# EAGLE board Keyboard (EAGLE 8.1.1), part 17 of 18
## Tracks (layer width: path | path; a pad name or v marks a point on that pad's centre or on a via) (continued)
S$17665
  Bottom 0: 136.24,76.22 136.19,76.17
S$17666
  Bottom 0: 136.19,76.17 136.01,75.89
S$17667
  Bottom 0: 136.01,75.89 135.93,75.58
S$17668
  Bottom 0: 135.93,75.58 135.93,75.25
S$17669
  Bottom 0: 135.93,75.25 136.01,74.94
S$17670
  Bottom 0: 136.01,74.94 136.11,74.79
S$17671
  Bottom 0: 136.11,74.79 133.86,77.04
S$17672
  Bottom 0: 133.86,77.04 133.81,77.09
S$17673
  Bottom 0: 133.81,77.09 133.75,77.12
S$17674
  Bottom 0: 133.75,77.12 133.68,77.15
S$17675
  Bottom 0: 133.68,77.15 133.61,77.17
S$17676
  Bottom 0: 133.61,77.17 133.55,77.17
S$17677
  Bottom 0: 133.55,77.17 123.08,77.17
S$17678
  Bottom 0: 123.08,77.17 123.01,77.17
S$17679
  Bottom 0: 123.01,77.17 122.94,77.15
S$17680
  Bottom 0: 122.94,77.15 122.88,77.13
S$17681
  Bottom 0: 122.88,77.13 122.82,77.09
S$17682
  Bottom 0: 122.82,77.09 122.77,77.05
S$17683
  Bottom 0: 122.77,77.05 120.27,74.55
S$17684
  Bottom 0: 120.27,74.55 118.87,74.55
S$17685
  Bottom 0: 131.47,79.17 131.77,79.23
S$17686
  Bottom 0: 131.77,79.23 132.03,79.39
S$17687
  Bottom 0: 132.03,79.39 132.24,79.61
S$17688
  Bottom 0: 132.24,79.61 132.37,79.88
S$17689
  Bottom 0: 132.37,79.88 132.41,80.18
S$17690
  Bottom 0: 132.41,80.18 132.37,80.48
S$17691
  Bottom 0: 132.37,80.48 132.24,80.75
S$17692
  Bottom 0: 132.24,80.75 132.03,80.97
S$17693
  Bottom 0: 132.03,80.97 131.77,81.12
S$17694
  Bottom 0: 131.77,81.12 131.47,81.19
S$17695
  Bottom 0: 131.47,81.19 131.17,81.17
S$17696
  Bottom 0: 131.17,81.17 130.89,81.06
S$17697
  Bottom 0: 130.89,81.06 130.65,80.87
S$17698
  Bottom 0: 130.65,80.87 130.48,80.62
S$17699
  Bottom 0: 130.48,80.62 130.39,80.33
S$17700
  Bottom 0: 130.39,80.33 130.39,80.03
S$17701
  Bottom 0: 130.39,80.03 130.48,79.74
S$17702
  Bottom 0: 130.48,79.74 130.65,79.49
S$17703
  Bottom 0: 130.65,79.49 130.89,79.3
S$17704
  Bottom 0: 130.89,79.3 131.17,79.19
S$17705
  Bottom 0: 131.17,79.19 131.47,79.17
S$17706
  Bottom 0: 125.75,79.83 126.1,79.89
S$17707
  Bottom 0: 126.1,79.89 126.41,80.04
S$17708
  Bottom 0: 126.41,80.04 126.68,80.26
S$17709
  Bottom 0: 126.68,80.26 126.89,80.55
S$17710
  Bottom 0: 126.89,80.55 127.02,80.87
S$17711
  Bottom 0: 127.02,80.87 127.06,81.22
S$17712
  Bottom 0: 127.06,81.22 127.02,81.56
S$17713
  Bottom 0: 127.02,81.56 126.89,81.89
S$17714
  Bottom 0: 126.89,81.89 126.68,82.17
S$17715
  Bottom 0: 126.68,82.17 126.41,82.39
S$17716
  Bottom 0: 126.41,82.39 126.1,82.55
S$17717
  Bottom 0: 126.1,82.55 125.75,82.61
S$17718
  Bottom 0: 125.75,82.61 125.4,82.59
S$17719
  Bottom 0: 125.4,82.59 125.07,82.48
S$17720
  Bottom 0: 125.07,82.48 124.78,82.29
S$17721
  Bottom 0: 124.78,82.29 124.54,82.04
S$17722
  Bottom 0: 124.54,82.04 124.37,81.73
S$17723
  Bottom 0: 124.37,81.73 124.28,81.39
S$17724
  Bottom 0: 124.28,81.39 124.28,81.04
S$17725
  Bottom 0: 124.28,81.04 124.37,80.7
S$17726
  Bottom 0: 124.37,80.7 124.54,80.39
S$17727
  Bottom 0: 124.54,80.39 124.78,80.14
S$17728
  Bottom 0: 124.78,80.14 125.07,79.95
S$17729
  Bottom 0: 125.07,79.95 125.4,79.84
S$17730
  Bottom 0: 125.4,79.84 125.75,79.83
S$17731
  Bottom 0: 121.86,81.47 122.3,81.52
S$17732
  Bottom 0: 122.3,81.52 122.73,81.64
S$17733
  Bottom 0: 122.73,81.64 123.13,81.86
S$17734
  Bottom 0: 123.13,81.86 123.47,82.14
S$17735
  Bottom 0: 123.47,82.14 123.76,82.49
S$17736
  Bottom 0: 123.76,82.49 123.97,82.88
S$17737
  Bottom 0: 123.97,82.88 124.1,83.31
S$17738
  Bottom 0: 124.1,83.31 124.14,83.76
S$17739
  Bottom 0: 124.14,83.76 124.1,84.2
S$17740
  Bottom 0: 124.1,84.2 123.97,84.63
S$17741
  Bottom 0: 123.97,84.63 123.76,85.03
S$17742
  Bottom 0: 123.76,85.03 123.47,85.37
S$17743
  Bottom 0: 123.47,85.37 123.13,85.66
S$17744
  Bottom 0: 123.13,85.66 122.73,85.87
S$17745
  Bottom 0: 122.73,85.87 122.3,86
S$17746
  Bottom 0: 122.3,86 121.86,86.04
S$17747
  Bottom 0: 121.86,86.04 121.41,86
S$17748
  Bottom 0: 121.41,86 120.98,85.87
S$17749
  Bottom 0: 120.98,85.87 120.59,85.66
S$17750
  Bottom 0: 120.59,85.66 120.24,85.37
S$17751
  Bottom 0: 120.24,85.37 119.96,85.03
S$17752
  Bottom 0: 119.96,85.03 119.74,84.63
S$17753
  Bottom 0: 119.74,84.63 119.61,84.2
S$17754
  Bottom 0: 119.61,84.2 119.57,83.76
S$17755
  Bottom 0: 119.57,83.76 119.61,83.31
S$17756
  Bottom 0: 119.61,83.31 119.74,82.88
S$17757
  Bottom 0: 119.74,82.88 119.96,82.49
S$17758
  Bottom 0: 119.96,82.49 120.24,82.14
S$17759
  Bottom 0: 120.24,82.14 120.59,81.86
S$17760
  Bottom 0: 120.59,81.86 120.98,81.64
S$17761
  Bottom 0: 120.98,81.64 121.41,81.52
S$17762
  Bottom 0: 121.41,81.52 121.86,81.47
S$17763
  Bottom 0: 131.47,86.79 131.77,86.86
S$17764
  Bottom 0: 131.77,86.86 132.03,87.01
S$17765
  Bottom 0: 132.03,87.01 132.24,87.23
S$17766
  Bottom 0: 132.24,87.23 132.37,87.5
S$17767
  Bottom 0: 132.37,87.5 132.41,87.8
S$17768
  Bottom 0: 132.41,87.8 132.37,88.1
S$17769
  Bottom 0: 132.37,88.1 132.24,88.37
S$17770
  Bottom 0: 132.24,88.37 132.03,88.59
S$17771
  Bottom 0: 132.03,88.59 131.77,88.75
S$17772
  Bottom 0: 131.77,88.75 131.47,88.81
S$17773
  Bottom 0: 131.47,88.81 131.17,88.79
S$17774
  Bottom 0: 131.17,88.79 130.89,88.68
S$17775
  Bottom 0: 130.89,88.68 130.65,88.49
S$17776
  Bottom 0: 130.65,88.49 130.48,88.24
S$17777
  Bottom 0: 130.48,88.24 130.39,87.95
S$17778
  Bottom 0: 130.39,87.95 130.39,87.65
S$17779
  Bottom 0: 130.39,87.65 130.48,87.36
S$17780
  Bottom 0: 130.48,87.36 130.65,87.11
S$17781
  Bottom 0: 130.65,87.11 130.89,86.92
S$17782
  Bottom 0: 130.89,86.92 131.17,86.81
S$17783
  Bottom 0: 131.17,86.81 131.47,86.79
S$17784
  Bottom 0: 174.03,75.35 172.15,77.23
S$17785
  Bottom 0: 172.15,77.23 172.09,77.27
S$17786
  Bottom 0: 172.09,77.27 172.03,77.31
S$17787
  Bottom 0: 172.03,77.31 171.97,77.34
S$17788
  Bottom 0: 171.97,77.34 171.91,77.36
S$17789
  Bottom 0: 171.91,77.36 171.83,77.36
S$17790
  Bottom 0: 171.83,77.36 168.25,77.36
S$17791
  Bottom 0: 168.25,77.36 165.01,80.6
S$17792
  Bottom 0: 165.01,80.6 165.12,80.87
S$17793
  Bottom 0: 165.12,80.87 165.16,81.22
S$17794
  Bottom 0: 165.16,81.22 165.12,81.56
S$17795
  Bottom 0: 165.12,81.56 164.99,81.89
S$17796
  Bottom 0: 164.99,81.89 164.78,82.17
S$17797
  Bottom 0: 164.78,82.17 164.51,82.39
S$17798
  Bottom 0: 164.51,82.39 164.2,82.55
S$17799
  Bottom 0: 164.2,82.55 163.85,82.61
S$17800
  Bottom 0: 163.85,82.61 163.5,82.59
S$17801
  Bottom 0: 163.5,82.59 163.17,82.48
S$17802
  Bottom 0: 163.17,82.48 162.88,82.29
S$17803
  Bottom 0: 162.88,82.29 162.64,82.04
S$17804
  Bottom 0: 162.64,82.04 162.56,81.9
S$17805
  Bottom 0: 162.56,81.9 162.56,81.99
S$17806
  Bottom 0: 162.56,81.99 162.88,82.31
S$17807
  Bottom 0: 162.88,82.31 162.94,82.38
S$17808
  Bottom 0: 162.94,82.38 162.99,82.45
S$17809
  Bottom 0: 162.99,82.45 163.03,82.53
S$17810
  Bottom 0: 163.03,82.53 163.04,82.62
S$17811
  Bottom 0: 163.04,82.62 163.05,82.71
S$17812
  Bottom 0: 163.05,82.71 163.05,87.58
S$17813
  Bottom 0: 163.05,87.58 163.04,87.67
S$17814
  Bottom 0: 163.04,87.67 163.03,87.76
S$17815
  Bottom 0: 163.03,87.76 162.99,87.84
S$17816
  Bottom 0: 162.99,87.84 162.94,87.92
S$17817
  Bottom 0: 162.94,87.92 162.88,87.98
S$17818
  Bottom 0: 162.88,87.98 162.33,88.54
S$17819
  Bottom 0: 162.33,88.54 162.37,88.84
S$17820
  Bottom 0: 162.37,88.84 162.32,89.16
S$17821
  Bottom 0: 162.32,89.16 162.19,89.46
S$17822
  Bottom 0: 162.19,89.46 162.01,89.65
S$17823
  Bottom 0: 162.01,89.65 176.59,89.65
S$17824
  Bottom 0: 176.59,89.65 176.59,87.95
S$17825
  Bottom 0: 176.59,87.95 176.6,87.87
S$17826
  Bottom 0: 176.6,87.87 176.64,87.8
S$17827
  Bottom 0: 176.64,87.8 176.7,87.74
S$17828
  Bottom 0: 176.7,87.74 176.77,87.7
S$17829
  Bottom 0: 176.77,87.7 176.85,87.69
S$17830
  Bottom 0: 176.85,87.69 177.24,87.69
S$17831
  Bottom 0: 177.24,87.69 174.62,85.08
S$17832
  Bottom 0: 174.62,85.08 174.58,85.03
S$17833
  Bottom 0: 174.58,85.03 174.54,84.97
S$17834
  Bottom 0: 174.54,84.97 174.51,84.91
S$17835
  Bottom 0: 174.51,84.91 174.5,84.84
S$17836
  Bottom 0: 174.5,84.84 174.49,84.77
S$17837
  Bottom 0: 174.49,84.77 174.49,76.36
S$17838
  Bottom 0: 174.49,76.36 174.29,76.17
S$17839
  Bottom 0: 174.29,76.17 174.12,75.89
S$17840
  Bottom 0: 174.12,75.89 174.03,75.58
S$17841
  Bottom 0: 174.03,75.58 174.03,75.35
S$17842
  Bottom 0: 169.24,78.25 169.76,78.25
S$17843
  Bottom 0: 169.76,78.25 170.27,78.34
S$17844
  Bottom 0: 170.27,78.34 170.76,78.5
S$17845
  Bottom 0: 170.76,78.5 171.21,78.75
S$17846
  Bottom 0: 171.21,78.75 171.62,79.07
S$17847
  Bottom 0: 171.62,79.07 171.98,79.45
S$17848
  Bottom 0: 171.98,79.45 172.26,79.88
S$17849
  Bottom 0: 172.26,79.88 172.47,80.36
S$17850
  Bottom 0: 172.47,80.36 172.6,80.86
S$17851
  Bottom 0: 172.6,80.86 172.64,81.37
S$17852
  Bottom 0: 172.64,81.37 172.6,81.89
S$17853
  Bottom 0: 172.6,81.89 172.47,82.39
S$17854
  Bottom 0: 172.47,82.39 172.26,82.87
S$17855
  Bottom 0: 172.26,82.87 171.98,83.3
S$17856
  Bottom 0: 171.98,83.3 171.62,83.68
S$17857
  Bottom 0: 171.62,83.68 171.21,84
S$17858
  Bottom 0: 171.21,84 170.76,84.24
S$17859
  Bottom 0: 170.76,84.24 170.27,84.41
S$17860
  Bottom 0: 170.27,84.41 169.76,84.5
S$17861
  Bottom 0: 169.76,84.5 169.24,84.5
S$17862
  Bottom 0: 169.24,84.5 168.74,84.41
S$17863
  Bottom 0: 168.74,84.41 168.24,84.24
S$17864
  Bottom 0: 168.24,84.24 167.79,84
S$17865
  Bottom 0: 167.79,84 167.38,83.68
S$17866
  Bottom 0: 167.38,83.68 167.03,83.3
S$17867
  Bottom 0: 167.03,83.3 166.74,82.87
S$17868
  Bottom 0: 166.74,82.87 166.53,82.39
S$17869
  Bottom 0: 166.53,82.39 166.41,81.89
S$17870
  Bottom 0: 166.41,81.89 166.37,81.37
S$17871
  Bottom 0: 166.37,81.37 166.41,80.86
S$17872
  Bottom 0: 166.41,80.86 166.53,80.36
S$17873
  Bottom 0: 166.53,80.36 166.74,79.88
S$17874
  Bottom 0: 166.74,79.88 167.03,79.45
S$17875
  Bottom 0: 167.03,79.45 167.38,79.07
S$17876
  Bottom 0: 167.38,79.07 167.79,78.75
S$17877
  Bottom 0: 167.79,78.75 168.24,78.5
S$17878
  Bottom 0: 168.24,78.5 168.74,78.34
S$17879
  Bottom 0: 168.74,78.34 169.24,78.25
S$17880
  Bottom 0: 322.05,75.88 321.98,76.03
S$17881
  Bottom 0: 321.98,76.03 321.77,76.29
S$17882
  Bottom 0: 321.77,76.29 321.51,76.48
S$17883
  Bottom 0: 321.51,76.48 321.2,76.58
S$17884
  Bottom 0: 321.2,76.58 320.88,76.6
S$17885
  Bottom 0: 320.88,76.6 320.56,76.54
S$17886
  Bottom 0: 320.56,76.54 320.27,76.39
S$17887
  Bottom 0: 320.27,76.39 320.09,76.22
S$17888
  Bottom 0: 320.09,76.22 320.09,79.82
S$17889
  Bottom 0: 320.09,79.82 320.24,79.81
S$17890
  Bottom 0: 320.24,79.81 320.55,79.86
S$17891
  Bottom 0: 320.55,79.86 320.65,79.83
S$17892
  Bottom 0: 320.65,79.83 321,79.81
S$17893
  Bottom 0: 321,79.81 321.35,79.87
S$17894
  Bottom 0: 321.35,79.87 321.66,80.02
S$17895
  Bottom 0: 321.66,80.02 321.93,80.25
S$17896
  Bottom 0: 321.93,80.25 322.05,80.41
S$17897
  Bottom 0: 322.05,80.41 322.05,75.88
S$17898
  Bottom 0: 223.34,79.41 222.16,80.6
S$17899
  Bottom 0: 222.16,80.6 222.27,80.87
S$17900
  Bottom 0: 222.27,80.87 222.31,81.22
S$17901
  Bottom 0: 222.31,81.22 222.27,81.56
S$17902
  Bottom 0: 222.27,81.56 222.14,81.89
S$17903
  Bottom 0: 222.14,81.89 221.93,82.17
S$17904
  Bottom 0: 221.93,82.17 221.66,82.39
S$17905
  Bottom 0: 221.66,82.39 221.35,82.55
S$17906
  Bottom 0: 221.35,82.55 221,82.61
S$17907
  Bottom 0: 221,82.61 220.65,82.59
S$17908
  Bottom 0: 220.65,82.59 220.32,82.48
S$17909
  Bottom 0: 220.32,82.48 220.03,82.29
S$17910
  Bottom 0: 220.03,82.29 219.79,82.04
S$17911
  Bottom 0: 219.79,82.04 219.79,82.06
S$17912
  Bottom 0: 219.79,82.06 220.03,82.31
S$17913
  Bottom 0: 220.03,82.31 220.09,82.38
S$17914
  Bottom 0: 220.09,82.38 220.14,82.45
S$17915
  Bottom 0: 220.14,82.45 220.18,82.53
S$17916
  Bottom 0: 220.18,82.53 220.19,82.62
S$17917
  Bottom 0: 220.19,82.62 220.2,82.71
S$17918
  Bottom 0: 220.2,82.71 220.2,87.58
S$17919
  Bottom 0: 220.2,87.58 220.19,87.66
S$17920
  Bottom 0: 220.19,87.66 220.18,87.75
S$17921
  Bottom 0: 220.18,87.75 220.14,87.84
S$17922
  Bottom 0: 220.14,87.84 220.09,87.91
S$17923
  Bottom 0: 220.09,87.91 220.03,87.98
S$17924
  Bottom 0: 220.03,87.98 219.48,88.54
S$17925
  Bottom 0: 219.48,88.54 219.52,88.84
S$17926
  Bottom 0: 219.52,88.84 219.49,89.05
S$17927
  Bottom 0: 219.49,89.05 226.21,82.32
S$17928
  Bottom 0: 226.21,82.32 226.21,81.09
S$17929
  Bottom 0: 226.21,81.09 226.14,81.06
S$17930
  Bottom 0: 226.14,81.06 225.91,80.88
S$17931
  Bottom 0: 225.91,80.88 225.74,80.63
S$17932
  Bottom 0: 225.74,80.63 225.64,80.34
S$17933
  Bottom 0: 225.64,80.34 225.64,80.03
S$17934
  Bottom 0: 225.64,80.03 225.74,79.74
S$17935
  Bottom 0: 225.74,79.74 225.91,79.49
S$17936
  Bottom 0: 225.91,79.49 226.01,79.41
S$17937
  Bottom 0: 226.01,79.41 223.34,79.41
S$17938
  Bottom 0.635: 284.09,74.83 284.09,60.85
S$17939
  Bottom 0.635: 284.09,60.85 291.67,53.27
S$17940
  Bottom 0.635: 276.67,22.46 276.67,23.03
S$17941
  Bottom 0.635: 284.99,22.81 284.99,15.92
S$17942
  Bottom 0.635: 284.99,15.92 283.31,14.24
S$17943
  Bottom 0.635: 283.31,14.24 282.44,14.24
S$17944
  Bottom 0.635: 282.44,14.24 276.67,20.02
S$17945
  Bottom 0.635: 276.67,20.02 276.67,22.46
S$17946
  Bottom 0.635: 275.4,22.46 276.67,22.46
S$17947
  Bottom 0.635: 275.4,22.46 275.4,21.32
S$17948
  Bottom 0.635: 275.4,23.03 275.4,22.46
S$17949
  Bottom 0.635: 274.13,23.03 274.13,21.32
S$17950
  Bottom 0.635: 274.13,21.32 275.4,21.32
S$17951
  Bottom 0.635: 289.13,38.03 287.6,39.56
S$17952
  Bottom 0.635: 287.6,39.56 285.93,39.56
S$17953
  Bottom 0.635: 285.93,39.56 285.14,38.78
S$17954
  Bottom 0.635: 285.14,38.78 285.14,35.23
S$17955
  Bottom 0.635: 285.14,35.23 286.46,33.91
S$17956
  Bottom 0.635: 286.46,33.91 286.46,24.28
S$17957
  Bottom 0.635: 286.46,24.28 284.99,22.81
S$17958
  Bottom 0.635: 291.67,53.27 291.81,53.13
S$17959
  Bottom 0.635: 291.81,53.13 291.81,40.71
S$17960
  Bottom 0.635: 291.81,40.71 289.13,38.03
S$17961
  Bottom 0.635: 284.09,74.83 285.37,74.83
S$17962
  Bottom 0.635: 283.78,74.83 284.09,74.83
S$17963
  Bottom 0.635: 289.88,88.52 289.88,85.48
S$17964
  Bottom 0.635: 289.88,85.48 287.82,83.42
S$17965
  Bottom 0.635: 285.37,74.83 285.37,80.97
S$17966
  Bottom 0.635: 285.37,80.97 287.82,83.42
S$17967
  Bottom 0.381: 23.05,62.84 23.05,58
S$17968
  Bottom 0.381: 23.05,58 21.43,56.38
S$17969
  Bottom 0.381: 21.43,56.38 21.43,36.5
S$17970
  Bottom 0.381: 21.43,36.5 19.45,34.52
S$17971
  Bottom 0.381: 19.45,34.52 19.45,31.01
S$17972
  Bottom 0.381: 19.45,31.01 23.27,27.18
S$17973
  Bottom 0.381: 23.27,27.18 23.27,24.07
S$17974
  Bottom 0.381: 11.37,81.21 23.05,69.53
S$17975
  Bottom 0.381: 23.05,69.53 23.05,62.84
S$17976
  Bottom 0.381: 30.31,62.84 23.05,62.84
S$17977
  Bottom 0.381: 230.44,62.16 217.85,62.16
S$17978
  Bottom 0.381: 217.85,62.16 211.53,68.49
S$17979
  Bottom 0.381: 211.53,68.49 205.24,68.49
S$17980
  Bottom 0.381: 205.24,68.49 198.23,75.5
S$17981
  Bottom 0.381: 198.23,75.5 198.23,78.82
S$17982
  Bottom 0.381: 198.23,78.82 195.58,81.46
S$17983
  Bottom 0.381: 195.58,81.46 195.58,84.68
S$17984
  Bottom 0.381: 195.58,84.68 198.04,87.14
S$17985
  Bottom 0.381: 198.04,87.14 198.04,89.98
S$17986
  Bottom 0.381: 198.04,89.98 197.93,90.09
S$17987
  Bottom 0.381: 197.93,90.09 195.67,90.09
S$17988
  Bottom 0.381: 195.67,90.09 186.8,81.22
S$17989
  Bottom 0.381: 186.8,81.22 182.82,81.22
S$17990
  Bottom 0.381: 225.09,10.39 243.96,29.27
S$17991
  Bottom 0.381: 243.96,29.27 243.96,50.19
S$17992
  Bottom 0.381: 243.96,50.19 231.99,62.16
S$17993
  Bottom 0.381: 231.99,62.16 230.44,62.16
S$17994
  Bottom 0.381: 225.09,10.39 224.25,11.23
S$17995
  Bottom 0.381: 224.25,11.23 219.46,11.23
S$17996
  Bottom 0.381: 219.46,11.23 206.63,24.07
S$17997
  Bottom 0.381: 228.06,5.01 228.06,7.42
S$17998
  Bottom 0.381: 228.06,7.42 225.09,10.39
S$17999
  Bottom 0.381: 101.85,43.11 101.85,49.98
S$18000
  Bottom 0.381: 101.85,49.98 94.96,56.87
S$18001
  Bottom 0.381: 94.96,56.87 90.32,56.87
S$18002
  Bottom 0.381: 90.32,56.87 87.39,59.8
S$18003
  Bottom 0.381: 206.63,24.07 208.01,25.45
S$18004
  Bottom 0.381: 208.01,25.45 208.01,41.25
S$18005
  Bottom 0.381: 208.01,41.25 201.14,48.12
S$18006
  Bottom 0.381: 30.42,81.21 24.39,81.21
S$18007
  Bottom 0.381: 24.39,81.21 22.5,79.33
S$18008
  Bottom 0.381: 22.5,79.33 22.5,77.87
S$18009
  Bottom 0.381: 22.5,77.87 25.14,75.23
S$18010
  Bottom 0.381: 25.14,75.23 25.14,68.47
S$18011
  Bottom 0.381: 25.14,68.47 29.97,63.64
S$18012
  Bottom 0.381: 29.97,63.64 29.98,63.65
S$18013
  Bottom 0.381: 29.98,63.65 30.64,63.65
S$18014
  Bottom 0.381: 30.64,63.65 31.11,63.18
S$18015
  Bottom 0.381: 31.11,63.18 31.11,62.51
S$18016
  Bottom 0.381: 31.11,62.51 31.1,62.51
S$18017
  Bottom 0.381: 31.1,62.51 31.3,62.3
S$18018
  Bottom 0.381: 31.3,62.3 33.06,62.3
S$18019
  Bottom 0.381: 33.06,62.3 41.18,54.18
S$18020
  Bottom 0.381: 41.18,54.18 40.9,53.9
S$18021
  Bottom 0.381: 40.9,53.9 40.9,49.1
S$18022
  Bottom 0.381: 40.9,49.1 36.84,45.04
S$18023
  Bottom 0.381: 36.84,45.04 36.84,39.84
S$18024
  Bottom 0.381: 36.84,39.84 46.75,29.93
S$18025
  Bottom 0.381: 46.75,29.93 50.49,29.93
S$18026
  Bottom 0.381: 50.49,29.93 54.23,26.2
S$18027
  Bottom 0.381: 54.23,26.2 54.23,24.07
S$18028
  Bottom 0.381: 41.18,54.18 43.28,56.28
S$18029
  Bottom 0.381: 43.28,56.28 72.4,56.28
S$18030
  Bottom 0.381: 72.4,56.28 74.52,58.39
S$18031
  Bottom 0.381: 248.65,36.62 248.65,19.02
S$18032
  Bottom 0.381: 248.65,19.02 245.54,15.91
S$18033
  Bottom 0.381: 245.54,15.91 245.54,11.47
S$18034
  Bottom 0.381: 245.54,11.47 246.21,10.8
S$18035
  Bottom 0.381: 246.21,10.8 248.34,10.8
S$18036
  Bottom 0.381: 248.34,10.8 251.88,7.26
S$18037
  Bottom 0.381: 251.88,7.26 251.88,5.01
S$18038
  Bottom 0.381: 258.57,55.84 248.65,45.92
S$18039
  Bottom 0.381: 248.65,45.92 248.65,36.62
S$18040
  Bottom 0.381: 258.57,55.84 261.87,52.54
S$18041
  Bottom 0.381: 261.87,52.54 279.47,52.54
S$18042
  Bottom 0.381: 279.47,52.54 281.36,54.43
S$18043
  Bottom 0.381: 281.36,54.43 282.4,54.43
S$18044
  Bottom 0.381: 74.52,58.39 74.52,58.64
S$18045
  Bottom 0.381: 74.52,58.64 78.04,62.16
S$18046
  Bottom 0.381: 81.73,45.79 81.73,51.17
S$18047
  Bottom 0.381: 81.73,51.17 74.52,58.39
S$18048
  Bottom 0.381: 258.57,55.84 253.28,61.13
S$18049
  Bottom 0.381: 253.28,61.13 250.52,61.13
S$18050
  Bottom 0.381: 250.52,61.13 249.49,62.16
S$18051
  Bottom 0.381: 249.49,62.16 241.63,62.16
S$18052
  Bottom 0.381: 241.63,62.16 235.93,67.86
S$18053
  Bottom 0.381: 235.93,67.86 219.61,67.86
S$18054
  Bottom 0.381: 219.61,67.86 213.66,73.81
S$18055
  Bottom 0.381: 213.66,73.81 212.67,73.81
S$18056
  Bottom 0.381: 212.67,73.81 209.28,77.21
S$18057
  Bottom 0.381: 209.28,77.21 205.87,77.21
S$18058
  Bottom 0.381: 205.87,77.21 201.87,81.21
S$18059
  Bottom 0.381: 225.68,24.07 225.68,31.66
S$18060
  Bottom 0.381: 225.68,31.66 223.92,33.42
S$18061
  Bottom 0.381: 223.92,33.42 223.92,36.87
S$18062
  Bottom 0.381: 139.95,43.11 140.71,43.11
S$18063
  Bottom 0.381: 140.71,43.11 147.98,50.38
S$18064
  Bottom 0.381: 147.98,50.38 147.98,56.3
S$18065
  Bottom 0.381: 147.98,56.3 150.48,58.8
S$18066
  Bottom 0.381: 150.48,58.8 150.48,61.23
S$18067
  Bottom 0.381: 150.48,61.23 153.63,64.38
S$18068
  Bottom 0.381: 153.63,64.38 153.63,68.95
S$18069
  Bottom 0.381: 85.43,62.16 74.68,72.92
S$18070
  Bottom 0.381: 74.68,72.92 74.68,74.86
S$18071
  Bottom 0.381: 77.19,24.06 77.19,32.81
S$18072
  Bottom 0.381: 77.19,32.81 85.43,41.04
S$18073
  Bottom 0.381: 85.43,41.04 85.43,62.16
S$18074
  Bottom 0.381: 281.31,53.24 261.67,33.61
S$18075
  Bottom 0.381: 261.67,33.61 261.67,24.33
S$18076
  Bottom 0.381: 261.67,24.33 261.4,24.06
S$18077
  Bottom 0.381: 273.3,62.16 252.72,62.16
S$18078
  Bottom 0.381: 252.72,62.16 247.12,67.75
S$18079
  Bottom 0.381: 247.12,67.75 237.6,67.75
S$18080
  Bottom 0.381: 237.6,67.75 226.39,78.97
S$18081
  Bottom 0.381: 226.39,78.97 223.16,78.97
S$18082
  Bottom 0.381: 223.16,78.97 220.92,81.21
S$18083
  Bottom 0.381: 97.09,62.16 85.43,62.16
S$18084
  Bottom 0.381: 282.06,5 277.23,5
S$18085
  Bottom 0.381: 277.23,5 270.83,11.39
S$18086
  Bottom 0.381: 270.83,11.39 270.83,14.63
S$18087
  Bottom 0.381: 270.83,14.63 261.4,24.06
S$18088
  Bottom 0.381: 124.25,58 124.25,60.96
S$18089
  Bottom 0.381: 124.25,60.96 108.49,76.73
S$18090
  Bottom 0.381: 108.49,76.73 104.85,76.73
S$18091
  Bottom 0.381: 104.85,76.73 102.22,74.1
S$18092
  Bottom 0.381: 102.22,74.1 98.07,74.1
S$18093
  Bottom 0.381: 98.07,74.1 95.44,76.73
S$18094
  Bottom 0.381: 95.44,76.73 92.06,76.73
S$18095
  Bottom 0.381: 92.06,76.73 87.57,81.21
S$18096
  Bottom 0.381: 113.96,22.9 113.96,31.13
S$18097
  Bottom 0.381: 113.96,31.13 124.25,41.41
S$18098
  Bottom 0.381: 124.25,41.41 124.25,58
S$18099
  Bottom 0.381: 124.25,58 131.03,58
S$18100
  Bottom 0.381: 131.03,58 135.19,62.16
S$18101
  Bottom 0.381: 287.22,56.36 275.81,67.77
S$18102
  Bottom 0.381: 275.81,67.77 267.81,67.77
S$18103
  Bottom 0.381: 267.81,67.77 266.96,68.61
S$18104
  Bottom 0.381: 266.96,68.61 266.96,79.64
S$18105
  Bottom 0.381: 266.96,79.64 268.54,81.21
S$18106
  Bottom 0.381: 178.05,43.11 178.05,50.67
S$18107
  Bottom 0.381: 178.05,50.67 172.72,56.01
S$18108
  Bottom 0.381: 111.38,24.06 111.38,10.24
S$18109
  Bottom 0.381: 111.38,10.24 105.09,3.95
S$18110
  Bottom 0.381: 301.83,53.27 292.74,44.18
S$18111
  Bottom 0.381: 292.74,44.18 292.74,41.6
S$18112
  Bottom 0.381: 320.53,5.38 320.15,5
S$18113
  Bottom 0.381: 320.92,62.15 322.28,60.78
S$18114
  Bottom 0.381: 322.28,60.78 322.28,7.13
S$18115
  Bottom 0.381: 322.28,7.13 320.53,5.38
S$18116
  Bottom 0.381: 320.91,5 320.53,5.38
S$18117
  Bottom 0.381: 204.25,5.01 206.44,2.82
S$18118
  Bottom 0.381: 206.44,2.82 215.8,2.82
S$18119
  Bottom 0.381: 215.8,2.82 217.05,4.07
S$18120
  Bottom 0.381: 217.05,4.07 224.34,4.07
S$18121
  Bottom 0.381: 224.34,4.07 224.97,3.43
S$18122
  Bottom 0.381: 224.97,3.43 228.62,3.43
S$18123
  Bottom 0.381: 228.62,3.43 246.78,21.59
S$18124
  Bottom 0.381: 246.78,21.59 246.78,49.38
S$18125
  Bottom 0.381: 212.45,63.23 207.81,67.86
S$18126
  Bottom 0.381: 207.81,67.86 205.07,67.86
S$18127
  Bottom 0.381: 205.07,67.86 200.22,72.72
S$18128
  Bottom 0.381: 200.22,72.72 194.71,72.72
S$18129
  Bottom 0.381: 194.71,72.72 190.67,76.76
S$18130
  Bottom 0.381: 190.67,76.76 181.09,76.76
S$18131
  Bottom 0.381: 181.09,76.76 178.43,74.1
S$18132
  Bottom 0.381: 178.43,74.1 174.65,74.1
S$18133
  Bottom 0.381: 174.65,74.1 171.83,76.91
S$18134
  Bottom 0.381: 171.83,76.91 168.07,76.91
S$18135
  Bottom 0.381: 168.07,76.91 163.77,81.22
S$18136
  Bottom 0.381: 212.45,63.23 223.69,51.99
S$18137
  Bottom 0.381: 223.69,51.99 240.96,51.99
S$18138
  Bottom 0.381: 240.96,51.99 243.16,49.79
S$18139
  Bottom 0.381: 211.39,62.16 212.45,63.23
S$18140
  Bottom 0.381: 82.8,43.11 84.16,44.47
S$18141
  Bottom 0.381: 84.16,44.47 84.16,58.18
S$18142
  Bottom 0.381: 84.16,58.18 75.22,67.12
S$18143
  Bottom 0.381: 75.22,67.12 44.89,67.12
S$18144
  Bottom 0.381: 44.89,67.12 39.94,62.17
S$18145
  Bottom 0.381: 204.25,5.01 204.25,11.95
S$18146
  Bottom 0.381: 204.25,11.95 196.74,19.45
S$18147
  Bottom 0.381: 196.74,19.45 192.19,19.45
S$18148
  Bottom 0.381: 192.19,19.45 187.58,24.07
S$18149
  Bottom 0.381: 266.16,43.11 273.33,50.28
S$18150
  Bottom 0.381: 116.14,62.16 116.14,64.42
S$18151
  Bottom 0.381: 116.14,64.42 112.7,67.86
S$18152
  Bottom 0.381: 112.7,67.86 110.61,67.86
S$18153
  Bottom 0.381: 110.61,67.86 105.64,72.84
S$18154
  Bottom 0.381: 105.64,72.84 105.64,73.03
S$18155
  Bottom 0.381: 104.63,27.61 107.56,30.54
S$18156
  Bottom 0.381: 107.56,30.54 107.56,33.11
S$18157
  Bottom 0.381: 107.56,33.11 110.82,36.38
S$18158
  Bottom 0.381: 110.82,36.38 112.63,36.38
S$18159
  Bottom 0.381: 112.63,36.38 116.97,40.72
S$18160
  Bottom 0.381: 116.97,40.72 116.97,42
S$18161
  Bottom 0.381: 116.97,42 122.28,47.31
S$18162
  Bottom 0.381: 122.28,47.31 122.28,56.03
S$18163
  Bottom 0.381: 122.28,56.03 116.14,62.16
S$18164
  Bottom 0.381: 283.86,51.96 283.95,51.96
S$18165
  Bottom 0.381: 283.86,51.96 283.86,56.89
S$18166
  Bottom 0.381: 283.86,56.89 273.54,67.21
S$18167
  Bottom 0.381: 273.54,67.21 265.36,67.21
S$18168
  Bottom 0.381: 265.36,67.21 265.02,67.55
S$18169
  Bottom 0.381: 265.02,67.55 259.51,67.55
S$18170
  Bottom 0.381: 259.51,67.55 259.04,67.08
S$18171
  Bottom 0.381: 259.04,67.08 255.53,67.08
S$18172
  Bottom 0.381: 255.53,67.08 251.21,71.4
S$18173
  Bottom 0.381: 251.21,71.4 249.08,71.4
S$18174
  Bottom 0.381: 249.08,71.4 239.97,80.52
S$18175
  Bottom 0.381: 239.97,80.52 239.97,81.21
S$18176
  Bottom 0.381: 271.53,37.76 271.53,39.63
S$18177
  Bottom 0.381: 271.53,39.63 283.86,51.96
S$18178
  Bottom 0.381: 159,43.11 159,51.53
S$18179
  Bottom 0.381: 159,51.53 155.37,55.17
S$18180
  Bottom 0.381: 300.58,5.52 300.13,5.07
S$18181
  Bottom 0.381: 300.13,5.07 290.26,5.07
S$18182
  Bottom 0.381: 290.26,5.07 285.16,10.17
S$18183
  Bottom 0.381: 285.16,10.17 277.1,10.17
S$18184
  Bottom 0.381: 277.1,10.17 271.53,15.74
S$18185
  Bottom 0.381: 271.53,15.74 271.53,37.76
S$18186
  Bottom 0.381: 271.53,37.76 268.2,37.76
S$18187
  Bottom 0.381: 300.58,5.52 301.1,5
S$18188
  Bottom 0.381: 301.11,24.05 300.58,23.52
S$18189
  Bottom 0.381: 300.58,23.52 300.58,5.52
S$18190
  Bottom 0.381: 301.1,62.15 301.1,55.08
S$18191
  Bottom 0.381: 301.1,55.08 299.29,53.27
S$18192
  Bottom 0.381: 154.24,62.16 154.56,62.48
S$18193
  Bottom 0.381: 154.56,62.48 154.56,69.15
S$18194
  Bottom 0.381: 154.56,69.15 149.32,74.39
S$18195
  Bottom 0.381: 149.32,74.39 145.73,74.39
S$18196
  Bottom 0.381: 145.73,74.39 145.33,73.98
S$18197
  Bottom 0.381: 145.33,73.98 136.29,73.98
S$18198
  Bottom 0.381: 136.29,73.98 133.55,76.73
S$18199
  Bottom 0.381: 133.55,76.73 123.08,76.73
S$18200
  Bottom 0.381: 123.08,76.73 120.46,74.1
S$18201
  Bottom 0.381: 120.46,74.1 117.12,74.1
S$18202
  Bottom 0.381: 117.12,74.1 113.94,77.28
S$18203
  Bottom 0.381: 113.94,77.28 110.55,77.28
S$18204
  Bottom 0.381: 110.55,77.28 106.62,81.22
S$18205
  Bottom 0.381: 122.5,20.09 115.91,26.69
S$18206
  Bottom 0.381: 115.91,26.69 115.91,31.06
S$18207
  Bottom 0.381: 115.91,31.06 123.8,38.96
S$18208
  Bottom 0.381: 123.8,38.96 138,38.96
S$18209
  Bottom 0.381: 138,38.96 149.31,50.27
S$18210
  Bottom 0.381: 149.31,50.27 149.31,56.45
S$18211
  Bottom 0.381: 149.31,56.45 154.24,61.37
S$18212
  Bottom 0.381: 154.24,61.37 154.24,62.16
S$18213
  Bottom 0.381: 37.56,5.02 26.05,5.02
S$18214
  Bottom 0.381: 26.05,5.02 22.58,1.54
S$18215
  Bottom 0.381: 22.58,1.54 17.22,1.54
S$18216
  Bottom 0.381: 17.22,1.54 16.48,2.28
S$18217
  Bottom 0.381: 16.48,2.28 16.48,4.42
S$18218
  Bottom 0.381: 16.48,4.42 9.93,10.98
S$18219
  Bottom 0.381: 9.93,10.98 9.93,34.53
S$18220
  Bottom 0.381: 9.93,34.53 18.51,43.12
S$18221
  Bottom 0.381: 122.5,20.09 105.56,3.15
S$18222
  Bottom 0.381: 105.56,3.15 57.11,3.15
S$18223
  Bottom 0.381: 57.11,3.15 54.6,5.67
S$18224
  Bottom 0.381: 54.6,5.67 38.21,5.67
S$18225
  Bottom 0.381: 38.21,5.67 37.56,5.02
S$18226
  Bottom 0.381: 122.5,20.09 122.72,19.88
S$18227
  Bottom 0.381: 122.72,19.88 126.24,19.88
S$18228
  Bottom 0.381: 126.24,19.88 130.43,24.06
S$18229
  Bottom 0.381: 197.1,43.12 197.1,45.24
S$18230
  Bottom 0.381: 197.1,45.24 193.53,48.81
S$18231
  Bottom 0.381: 193.53,48.81 191.43,48.81
S$18232
  Bottom 0.381: 191.43,48.81 189.1,51.14
S$18233
  Bottom 0.381: 189.1,51.14 189.1,51.36
S$18234
  Bottom 0.381: 301.86,81.2 304.37,78.69
S$18235
  Bottom 0.381: 304.37,78.69 304.37,53.27
S$18236
  Bottom 0.381: 158.44,62.41 157.97,61.94
S$18237
  Bottom 0.381: 157.97,61.94 157.39,61.94
S$18238
  Bottom 0.381: 157.39,61.94 150.09,54.64
S$18239
  Bottom 0.381: 150.09,54.64 150.09,48.2
S$18240
  Bottom 0.381: 150.09,48.2 144.5,42.6
S$18241
  Bottom 0.381: 144.5,42.6 144.5,38.51
S$18242
  Bottom 0.381: 144.5,38.51 145.95,37.06
S$18243
  Bottom 0.381: 144.72,81.22 144.72,80.58
S$18244
  Bottom 0.381: 144.72,80.58 158.44,66.85
S$18245
  Bottom 0.381: 158.44,66.85 158.44,62.41
S$18246
  Bottom 0.381: 158.44,62.41 158.6,62.26
S$18247
  Bottom 0.381: 158.6,62.26 170.78,62.26
S$18248
  Bottom 0.381: 170.78,62.26 172.22,63.71
S$18249
  Bottom 0.381: 172.22,63.71 175.9,63.71
S$18250
  Bottom 0.381: 175.9,63.71 177.3,62.3
S$18251
  Bottom 0.381: 177.3,62.3 192.34,62.3
S$18252
  Bottom 0.381: 63.76,43.11 55.07,43.11
S$18253
  Bottom 0.381: 55.07,43.11 46.46,51.72
S$18254
  Bottom 0.381: 46.46,51.72 46.46,54.45
S$18255
  Bottom 0.381: 147.85,19.9 147.85,25.27
S$18256
  Bottom 0.381: 147.85,25.27 148.32,25.73
S$18257
  Bottom 0.381: 148.32,25.73 148.32,33.35
S$18258
  Bottom 0.381: 148.32,33.35 147.62,34.04
S$18259
  Bottom 0.381: 147.62,34.04 147.62,36.47
S$18260
  Bottom 0.381: 147.62,36.47 148.19,37.04
S$18261
  Bottom 0.381: 192.34,62.3 192.34,62.17
S$18263
  Bottom 0.381: 235.2,43.12 225.15,43.12
S$18264
  Bottom 0.381: 225.15,43.12 199.51,68.75
S$18265
  Bottom 0.381: 199.51,68.75 199.51,68.98
S$18266
  Bottom 0.381: 199.51,68.98 198.61,69.89
S$18267
  Bottom 0.381: 198.61,69.89 197.39,69.89
S$18268
  Bottom 0.381: 197.39,69.89 192.34,64.84
S$18269
  Bottom 0.381: 192.34,64.84 192.34,62.3
S$18270
  Bottom 0.381: 147.85,19.9 147.7,19.9
S$18271
  Bottom 0.381: 147.7,19.9 132.81,5.01
S$18272
  Bottom 0.381: 168.53,24.06 164.36,19.9
S$18273
  Bottom 0.381: 164.36,19.9 147.85,19.9
S$18274
  Bottom 0.381: 157.64,62.74 157.64,66.86
S$18275
  Bottom 0.381: 157.64,66.86 147.78,76.72
S$18276
  Bottom 0.381: 147.78,76.72 142.8,76.72
S$18277
  Bottom 0.381: 142.8,76.72 138.11,81.42
S$18278
  Bottom 0.381: 173.29,62.16 169.11,57.98
S$18279
  Bottom 0.381: 169.11,57.98 156.25,57.98
S$18280
  Bottom 0.381: 156.25,57.98 154.48,56.22
S$18281
  Bottom 0.381: 154.48,56.22 154.48,54.92
S$18282
  Bottom 0.381: 154.48,54.92 157.85,51.55
S$18283
  Bottom 0.381: 157.85,51.55 157.85,44.76
S$18284
  Bottom 0.381: 157.85,44.76 157.43,44.33
S$18285
  Bottom 0.381: 157.43,44.33 157.43,43.2
S$18286
  Bottom 0.381: 157.43,43.2 152.31,38.09
S$18287
  Bottom 0.381: 152.31,38.09 150.79,38.09
S$18288
  Bottom 0.381: 150.79,38.09 148.18,35.48
S$18289
  Bottom 0.381: 148.18,35.48 148.18,34.32
S$18290
  Bottom 0.381: 148.18,34.32 149.48,33.03
S$18291
  Bottom 0.381: 149.48,33.03 149.48,24.07
S$18292
  Bottom 0.381: 216.15,43.12 216.15,45.24
S$18293
  Bottom 0.381: 216.15,45.24 213.34,48.06
S$18294
  Bottom 0.381: 213.34,48.06 206.34,48.06
S$18295
  Bottom 0.381: 206.34,48.06 197.36,57.03
S$18296
  Bottom 0.381: 197.36,57.03 178.43,57.03
S$18297
  Bottom 0.381: 178.43,57.03 173.29,62.16
S$18298
  Bottom 0.381: 306.91,53.27 305.91,54.27
S$18299
  Bottom 0.381: 305.91,54.27 305.91,69.6
S$18300
  Bottom 0.381: 305.91,69.6 306.85,70.54
S$18301
  Bottom 0.381: 306.85,70.54 309.44,70.54
S$18302
  Bottom 0.381: 309.44,70.54 311.57,68.41
S$18303
  Bottom 0.381: 311.57,68.41 318.94,68.41
S$18304
  Bottom 0.381: 318.94,68.41 319.65,69.12
S$18305
  Bottom 0.381: 319.65,69.12 319.65,80.7
S$18306
  Bottom 0.381: 319.65,80.7 320.15,81.2
S$18307
  Bottom 0.381: 70.58,18.76 70.58,14.23
S$18308
  Bottom 0.381: 70.58,14.23 61.37,5.02
S$18309
  Bottom 0.381: 44.7,43.12 51.31,36.51
S$18310
  Bottom 0.381: 51.31,36.51 65.97,36.51
S$18311
  Bottom 0.381: 65.97,36.51 69.46,33.02
S$18312
  Bottom 0.381: 69.46,33.02 69.46,30.86
S$18313
  Bottom 0.381: 69.46,30.86 71.93,28.38
S$18314
  Bottom 0.381: 71.93,28.38 71.93,25.54
S$18315
  Bottom 0.381: 71.93,25.54 70.58,24.2
S$18316
  Bottom 0.381: 70.58,24.2 70.58,18.76
S$18317
  Bottom 0.381: 198.07,68.75 224.27,42.55
S$18318
  Bottom 0.381: 224.27,42.55 232.91,42.55
S$18319
  Bottom 0.381: 232.91,42.55 233.86,41.6
S$18320
  Bottom 0.381: 233.86,41.6 235.85,41.6
S$18321
  Bottom 0.381: 235.85,41.6 242.62,48.37
S$18322
  Bottom 0.381: 242.62,48.37 242.62,48.87
S$18323
  Bottom 0.381: 64.71,68.75 63.84,67.88
S$18324
  Bottom 0.381: 63.84,67.88 46.52,67.88
S$18325
  Bottom 0.381: 46.52,67.88 45.66,68.75
S$18326
  Bottom 0.381: 102.81,68.75 102.36,68.3
S$18327
  Bottom 0.381: 102.36,68.3 84.21,68.3
S$18328
  Bottom 0.381: 84.21,68.3 83.76,68.75
S$18329
  Bottom 0.381: 140.91,68.75 140.57,68.41
S$18330
  Bottom 0.381: 140.57,68.41 122.21,68.41
S$18331
  Bottom 0.381: 122.21,68.41 121.87,68.75
S$18332
  Bottom 0.635: 303.52,17.49 303.52,30.17
S$18333
  Bottom 0.635: 303.52,30.17 301.91,31.78
S$18334
  Bottom 0.635: 301.91,31.78 301.91,34.94
S$18335
  Bottom 0.635: 44.71,53.99 44.71,54.01
S$18336
  Bottom 0.635: 44.71,54.01 46.17,55.47
S$18337
  Bottom 0.635: 46.17,55.47 62.27,55.47
S$18338
  Bottom 0.635: 62.27,55.47 63.76,53.98
S$18339
  Bottom 0.635: 68.52,75.42 68.89,75.78
S$18340
  Bottom 0.635: 68.89,75.78 75.31,75.78
S$18341
  Bottom 0.635: 75.31,75.78 78.05,73.04
S$18342
  Bottom 0.635: 12.2,49.24 1.6,38.64
S$18343
  Bottom 0.635: 1.6,38.64 1.6,13.74
S$18344
  Bottom 0.635: 16.57,49.24 12.2,49.24
S$18345
  Bottom 0.635: 12.2,49.24 12.04,49.39
S$18346
  Bottom 0.635: 12.04,49.39 12.04,60.73
S$18347
  Bottom 0.635: 12.04,60.73 16.13,64.81
S$18348
  Bottom 0.635: 16.13,64.81 16.13,73.04
S$18349
  Bottom 0.635: 163.78,75.42 170.93,75.42
S$18350
  Bottom 0.635: 170.93,75.42 173.31,73.04
S$18351
  Bottom 0.635: 249.51,73.04 251.42,73.04
S$18352
  Bottom 0.635: 251.42,73.04 253.81,70.66
S$18353
  Bottom 0.635: 301.91,73.04 301.91,75.42
S$18354
  Bottom 0.635: 320.96,73.04 320.96,75.42
S$18355
  Bottom 0.635: 182.84,75.42 189.99,75.42
S$18356
  Bottom 0.635: 189.99,75.42 192.36,73.04
S$18357
  Bottom 0.635: 173.31,73.04 180.46,73.04
S$18358
  Bottom 0.635: 180.46,73.04 182.84,75.42
S$18359
  Bottom 0.635: 16.13,73.04 13.74,73.04
S$18360
  Bottom 0.635: 13.74,73.04 11.37,75.42
S$18361
  Bottom 0.635: 17.32,53.98 17.5,53.8
S$18362
  Bottom 0.635: 17.5,53.8 17.5,50.16
S$18363
  Bottom 0.635: 17.5,50.16 16.57,49.24
S$18364
  Bottom 0.635: 17.32,37.31 20.26,40.25
S$18365
  Bottom 0.635: 20.26,40.25 20.26,45.55
S$18366
  Bottom 0.635: 20.26,45.55 16.57,49.24
S$18367
  Bottom 0.635: 168.55,34.94 168.26,34.94
S$18368
  Bottom 0.635: 168.26,34.94 160.77,42.43
S$18369
  Bottom 0.635: 177.98,33.07 170.41,33.07
S$18370
  Bottom 0.635: 170.41,33.07 168.55,34.94
S$18371
  Bottom 0.635: 160.77,42.43 153.28,34.94
S$18372
  Bottom 0.635: 153.28,34.94 149.49,34.94
S$18373
  Bottom 0.635: 159.02,53.99 160.77,52.24
S$18374
  Bottom 0.635: 160.77,52.24 160.77,42.43
S$18375
  Bottom 0.635: 61.38,15.89 61.38,13.12
S$18376
  Bottom 0.635: 61.38,13.12 58.55,10.29
S$18377
  Bottom 0.635: 58.55,10.29 43.16,10.29
S$18378
  Bottom 0.635: 43.16,10.29 42.09,11.36
S$18379
  Bottom 0.635: 54.23,34.94 58.49,30.68
S$18380
  Bottom 0.635: 58.49,30.68 58.49,18.77
S$18381
  Bottom 0.635: 58.49,18.77 61.38,15.89
S$18382
  Bottom 0.635: 266.19,53.99 270.95,53.99
S$18383
  Bottom 0.635: 270.95,53.99 277.86,60.89
S$18384
  Bottom 0.635: 82.81,53.99 82.81,45.56
S$18385
  Bottom 0.635: 82.81,45.56 79.22,41.97
S$18386
  Bottom 0.635: 79.22,41.97 78.98,41.97
S$18387
  Bottom 0.635: 125.68,75.35 132.89,75.35
S$18388
  Bottom 0.635: 132.89,75.35 135.2,73.04
S$18389
  Bottom 0.635: 116.15,73.04 123.37,73.04
S$18390
  Bottom 0.635: 123.37,73.04 125.68,75.35
S$18391
  Bottom 0.635: 125.68,75.35 125.68,75.42
S$18392
  Bottom 0.635: 78.98,41.97 66.97,53.98
S$18393
  Bottom 0.635: 66.97,53.98 63.76,53.98
S$18394
  Bottom 0.635: 73.28,34.94 78.98,40.63
S$18395
  Bottom 0.635: 78.98,40.63 78.98,41.97
S$18396
  Bottom 0.635: 39.94,73.04 37.57,75.42
S$18397
  Bottom 0.635: 37.57,75.42 30.42,75.42
S$18398
  Bottom 0.635: 49.47,75.42 47.1,73.04
S$18399
  Bottom 0.635: 47.1,73.04 39.94,73.04
S$18400
  Bottom 0.635: 230.23,30.41 228.08,28.27
S$18401
  Bottom 0.635: 228.08,28.27 228.08,15.88
S$18402
  Bottom 0.635: 225.7,34.94 230.23,30.41
S$18403
  Bottom 0.635: 230.23,30.41
S$18404
  Bottom 0.635: 59,73.05 56.63,75.42
S$18405
  Bottom 0.635: 56.63,75.42 49.47,75.42
S$18406
  Bottom 0.635: 87.58,75.42 85.2,73.04
S$18407
  Bottom 0.635: 85.2,73.04 78.05,73.04
S$18408
  Bottom 0.635: 97.1,73.04 94.72,75.42
S$18409
  Bottom 0.635: 94.72,75.42 87.58,75.42
S$18410
  Bottom 0.635: 301.91,15.89 303.52,17.49
S$18411
  Bottom 0.635: 303.52,17.49 319.36,17.49
S$18412
  Bottom 0.635: 319.36,17.49 320.96,15.89
S$18413
  Bottom 0.635: 104.09,73.04 97.1,73.04
S$18414
  Bottom 0.635: 206.65,34.94 206.65,26.86
S$18415
  Bottom 0.635: 206.65,26.86 204.27,24.48
S$18416
  Bottom 0.635: 204.27,24.48 204.27,15.88
S$18417
  Bottom 0.635: 195.49,52.35 206.65,41.19
S$18418
  Bottom 0.635: 206.65,41.19 206.65,34.94
S$18419
  Bottom 0.635: 106.63,75.42 104.25,73.04
S$18420
  Bottom 0.635: 104.25,73.04 104.09,73.04
S$18421
  Bottom 0.635: 101.86,53.98 104.09,56.22
S$18422
  Bottom 0.635: 104.09,56.22 104.09,73.04
S$18423
  Bottom 0.635: 103.5,52.35 101.86,53.98
S$18424
  Bottom 0.635: 195.49,52.35 197.12,53.98
S$18425
  Bottom 0.635: 179.71,52.35 195.49,52.35
S$18426
  Bottom 0.635: 95.83,34.65 103.5,42.31
S$18427
  Bottom 0.635: 103.5,42.31 103.5,52.35
S$18428
  Bottom 0.635: 103.5,52.35 119.28,52.35
S$18429
  Bottom 0.635: 119.28,52.35 120.91,53.99
S$18430
  Bottom 0.635: 179.71,52.35 178.07,53.98
S$18431
  Bottom 0.635: 178.41,33.3 178.41,36.6
S$18432
  Bottom 0.635: 178.41,36.6 179.71,37.9
S$18433
  Bottom 0.635: 179.71,37.9 179.71,52.35
S$18434
  Bottom 0.635: 95.83,34.65 95.54,34.94
S$18435
  Bottom 0.635: 95.54,34.94 92.34,34.94
S$18436
  Bottom 0.635: 107.47,23 95.83,34.65
S$18437
  Bottom 0.635: 177.98,33.07 178.18,33.07
S$18438
  Bottom 0.635: 178.18,33.07 178.41,33.3
S$18439
  Bottom 0.635: 178.41,33.3 185.96,33.3
S$18440
  Bottom 0.635: 185.96,33.3 187.6,34.94
S$18441
  Bottom 0.635: 272.86,28.03 272.86,26.32
S$18442
  Bottom 0.635: 274.13,28.03 274.13,26.32
S$18443
  Bottom 0.635: 275.4,28.03 275.4,26.32
S$18444
  Bottom 0.635: 276.67,28.03 276.67,26.32
S$18445
  Bottom 0.635: 276.67,26.32 277.58,25.41
S$18446
  Bottom 0.635: 277.58,25.41 277.58,21.16
S$18447
  Bottom 0.635: 277.58,21.16 282.86,15.88
S$18448
  Bottom 0.635: 276.67,26.32 275.4,26.32
S$18449
  Bottom 0.635: 274.13,26.32 272.86,26.32
S$18450
  Bottom 0.635: 275.4,26.32 274.13,26.32
S$18451
  Bottom 0.635: 111.39,34.94 111.39,26.71
S$18452
  Bottom 0.635: 111.39,26.71 107.68,23
S$18453
  Bottom 0.635: 107.68,23 107.47,23
S$18454
  Bottom 0.635: 106.61,7.43 107.47,8.3
S$18455
  Bottom 0.635: 107.47,8.3 107.47,23
S$18456
  Bottom 0.635: 177.98,7.51 177.98,33.07
S$18457
  Bottom 0.381: 145.68,49.7 145.41,49.44
S$18458
  Bottom 0.381: 145.41,49.44 126.89,49.44
S$18459
  Bottom 0.381: 126.89,49.44 126.62,49.7
S$18460
  Bottom 0.381: 240.94,49.7 240.63,49.39
S$18461
  Bottom 0.381: 240.63,49.39 222.2,49.39
S$18462
  Bottom 0.381: 222.2,49.39 221.89,49.7
S$18463
  Bottom 0.381: 299.29,38.03 301.08,36.24
S$18464
  Bottom 0.381: 301.08,36.24 302.45,36.24
S$18465
  Bottom 0.381: 302.45,36.24 304.4,34.3
S$18466
  Bottom 0.381: 304.4,34.3 304.4,30.6
S$18467
  Bottom 0.381: 258.8,5.88 260.02,7.1
S$18468
  Bottom 0.381: 260.02,7.1 260.02,23.19
S$18469
  Bottom 0.381: 260.02,23.19 259.81,23.41
S$18470
  Bottom 0.381: 259.81,23.41 259.81,24.85
S$18471
  Bottom 0.381: 259.81,24.85 260.87,25.91
S$18472
  Bottom 0.381: 260.87,25.91 260.87,27.64
S$18473
  Bottom 0.381: 114.25,15.88 115.58,15.88
S$18474
  Bottom 0.381: 115.58,15.88 117.43,17.74
S$18475
  Bottom 0.381: 44.47,11.6 43.39,12.67
S$18476
  Bottom 0.381: 43.39,12.67 37.02,12.67
S$18477
  Bottom 0.381: 37.02,12.67 34.39,10.05
S$18478
  Bottom 0.381: 34.39,10.05 29.78,10.05
S$18479
  Bottom 0.381: 29.78,10.05 22.52,2.78
S$18480
  Bottom 0.381: 22.52,2.78 17.8,2.78
S$18481
  Bottom 0.381: 185.69,15.88 185.69,24.45
S$18482
  Bottom 0.381: 185.69,24.45 191.89,30.65
S$18483
  Bottom 0.381: 191.89,30.65 193.31,30.65
S$18484
  Bottom 0.381: 291.67,38.03 293.26,36.44
S$18485
  Bottom 0.381: 293.26,36.44 296.41,36.44
S$18486
  Bottom 0.381: 296.41,36.44 299.69,33.16
S$18487
  Bottom 0.381: 307.63,68.75 309.22,67.15
S$18488
  Bottom 0.381: 309.22,67.15 309.22,61.02
S$18489
  Bottom 0.381: 309.22,61.02 315.9,54.33
S$18490
  Bottom 0.381: 315.9,54.33 315.9,47.03
S$18491
  Bottom 0.381: 315.9,47.03 306.91,38.03
S$18492
  Bottom 0.381: 69.47,49.7 69.16,49.39
S$18493
  Bottom 0.381: 69.16,49.39 50.73,49.39
S$18494
  Bottom 0.381: 50.73,49.39 50.42,49.7
S$18495
  Bottom 0.381: 189.74,87.8 187.45,90.09
S$18496
  Bottom 0.381: 187.45,90.09 81.04,90.09
S$18497
  Bottom 0.381: 81.04,90.09 59.38,68.44
S$18498
  Bottom 0.381: 59.38,68.44 52.93,68.44
S$18499
  Bottom 0.381: 52.93,68.44 51.49,69.88
S$18500
  Bottom 0.381: 51.49,69.88 39.45,69.88
S$18501
  Bottom 0.381: 39.45,69.88 37.98,68.41
S$18502
  Bottom 0.381: 37.98,68.41 26.95,68.41
S$18503
  Bottom 0.381: 26.95,68.41 26.61,68.75
S$18504
  Bottom 0.381: 311.99,38.03 316.47,42.51
S$18505
  Bottom 0.381: 316.47,42.51 316.47,60.7
S$18506
  Bottom 0.381: 316.47,60.7 309.78,67.38
S$18507
  Bottom 0.381: 309.78,67.38 309.78,68.42
S$18508
  Bottom 0.381: 309.78,68.42 308.22,69.98
S$18509
  Bottom 0.381: 308.22,69.98 307.08,69.98
S$18510
  Bottom 0.381: 307.08,69.98 306.47,69.37
S$18511
  Bottom 0.381: 306.47,69.37 306.47,67.46
S$18512
  Bottom 0.381: 306.47,67.46 306.71,67.22
S$18513
  Bottom 0.381: 244.52,87.8 244.33,87.8
S$18514
  Bottom 0.381: 244.33,87.8 238.39,81.86
S$18515
  Bottom 0.381: 238.39,81.86 238.39,79.34
S$18516
  Bottom 0.381: 238.39,79.34 245.68,72.05
S$18517
  Bottom 0.381: 245.68,72.05 245.68,69.13
S$18518
  Bottom 0.381: 245.68,69.13 246.49,68.32
S$18519
  Bottom 0.381: 246.49,68.32 248.85,68.32
S$18520
  Bottom 0.381: 248.85,68.32 254.2,62.97
S$18521
  Bottom 0.381: 287.39,80.66 286.25,79.53
S$18522
  Bottom 0.381: 286.25,79.53 286.25,65.37
S$18523
  Bottom 0.381: 286.25,65.37 285.27,64.39
S$18524
  Bottom 0.381: 281.42,30.43 281.42,39.88
S$18525
  Bottom 0.381: 281.42,39.88 290.88,49.34
S$18526
  Bottom 0.381: 290.88,49.34 290.88,48.83
S$18527
  Bottom 0.381: 314.53,38.03 317.16,40.66
S$18528
  Bottom 0.381: 317.16,40.66 317.16,61.32
S$18529
  Bottom 0.381: 317.16,61.32 322.49,66.65
S$18530
  Bottom 0.381: 322.49,66.65 322.49,81.77
S$18531
  Bottom 0.381: 322.49,81.77 317.69,86.57
S$18532
  Bottom 0.381: 296.78,88.82 300.5,85.1
S$18533
  Bottom 0.381: 300.5,85.1 300.5,82.77
S$18534
  Bottom 0.381: 300.5,82.77 299.59,81.85
S$18535
  Bottom 0.381: 299.59,81.85 299.59,79.98
S$18536
  Bottom 0.381: 299.59,79.98 300.59,78.98
S$18537
  Bottom 0.381: 300.59,78.98 300.59,69.22
S$18538
  Bottom 0.381: 300.59,69.22 299.75,68.39
S$18539
  Bottom 0.381: 299.75,68.39 295.06,68.39
S$18540
  Bottom 0.381: 295.06,68.39 292.94,70.52
S$18541
  Bottom 0.381: 292.94,70.52 292.94,74.06
S$18542
  Bottom 0.381: 292.94,74.06 294.29,75.42
S$18543
  Bottom 0.635: 266,88.83 266.57,88.83
S$18544
  Bottom 0.635: 266.57,88.83 276.19,79.21
S$18545
  Bottom 0.635: 276.19,79.21 276.19,76.81
S$18546
  Bottom 0.635: 317.61,88.82 317.61,88.2
S$18547
  Bottom 0.635: 317.61,88.2 316.55,87.14
S$18548
  Bottom 0.635: 316.55,87.14 316.09,87.14
S$18549
  Bottom 0.635: 316.09,87.14 313.72,84.76
S$18550
  Bottom 0.635: 313.72,84.76 313.72,82.74
S$18551
  Bottom 0.635: 313.72,82.74 318.38,78.08
S$18552
  Bottom 0.635: 318.38,78.08 318.38,69.77
S$18553
  Bottom 0.635: 299.32,88.82 300.71,90.21
S$18554
  Bottom 0.635: 300.71,90.21 316.88,90.21
S$18555
  Bottom 0.635: 316.88,90.21 317.61,89.47
S$18556
  Bottom 0.635: 317.61,89.47 317.61,88.82
S$18557
  Bottom 0.635: 146.94,31.69 146.94,41.21
S$18558
  Bottom 0.635: 146.94,41.21 156.46,50.73
S$18559
  Bottom 0.635: 161.23,88.84 162.48,87.58
S$18560
  Bottom 0.635: 162.48,87.58 162.48,82.71
S$18561
  Bottom 0.635: 162.48,82.71 161.99,82.22
S$18562
  Bottom 0.635: 161.99,82.22 161.99,73.36
S$18563
  Bottom 0.635: 161.99,73.36 166.96,68.4
S$18564
  Bottom 0.635: 166.96,68.4 169.37,68.4
S$18565
  Bottom 0.635: 169.37,68.4 170.75,69.78
S$18566
  Bottom 0.635: 199.33,88.83 200.58,87.57
S$18567
  Bottom 0.635: 200.58,87.57 200.58,82.7
S$18568
  Bottom 0.635: 200.58,82.7 200.17,82.29
S$18569
  Bottom 0.635: 200.17,82.29 200.17,80.48
S$18570
  Bottom 0.635: 200.17,80.48 208.85,71.8
S$18571
  Bottom 0.635: 208.85,71.8 208.85,69.78
S$18572
  Bottom 0.635: 146.68,64.76 141.39,70.05
S$18573
  Bottom 0.635: 141.39,70.05 132.92,70.05
S$18574
  Bottom 0.635: 132.92,70.05 132.65,69.78
S$18575
  Bottom 0.635: 146.68,64.76 151.7,69.78
S$18576
  Bottom 0.635: 137.41,50.73 137.41,55.5
S$18577
  Bottom 0.635: 137.41,55.5 146.68,64.76
S$18578
  Bottom 0.635: 218.38,88.83 219.63,87.57
S$18579
  Bottom 0.635: 219.63,87.57 219.63,82.7
S$18580
  Bottom 0.635: 219.63,82.7 219.22,82.29
S$18581
  Bottom 0.635: 219.22,82.29 219.22,80.58
S$18582
  Bottom 0.635: 219.22,80.58 227.9,71.9
S$18583
  Bottom 0.635: 227.9,71.9 227.9,69.78
S$18584
  Bottom 0.635: 8.83,88.83 10.09,87.57
S$18585
  Bottom 0.635: 10.09,87.57 10.09,82.7
S$18586
  Bottom 0.635: 10.09,82.7 9.73,82.34
S$18587
  Bottom 0.635: 9.73,82.34 9.73,74.31
S$18588
  Bottom 0.635: 9.73,74.31 13.59,70.45
S$18589
  Bottom 0.635: 13.59,70.45 13.59,69.79
S$18590
  Bottom 0.635: 91.31,42.91 89.79,41.38
S$18591
  Bottom 0.635: 89.79,41.38 89.79,31.68
S$18592
  Bottom 0.635: 91.31,42.91 86.74,47.47
S$18593
  Bottom 0.635: 86.74,47.47 86.74,49.22
S$18594
  Bottom 0.635: 99.31,50.73 91.49,42.91
S$18595
  Bottom 0.635: 91.49,42.91 91.31,42.91
S$18596
  Bottom 0.635: 20.73,31.69 26.98,25.43
S$18597
  Bottom 0.635: 26.98,25.43 35.02,17.4
S$18598
  Bottom 0.635: 26.98,25.43 14.19,12.63
S$18599
  Bottom 0.635: 14.19,12.63 11.21,12.63
S$18600
  Bottom 0.635: 55.99,17.4 35.02,17.4
S$18601
  Bottom 0.635: 58.83,12.64 55.99,15.48
S$18602
  Bottom 0.635: 55.99,15.48 55.99,17.4
S$18603
  Bottom 0.635: 51.69,31.69 55.99,27.38
S$18604
  Bottom 0.635: 55.99,27.38 55.99,17.4
S$18605
  Bottom 0.635: 35.02,17.4 35.02,12.64
S$18606
  Bottom 0.635: 170.3,27.38 173.5,27.38
S$18607
  Bottom 0.635: 173.5,27.38 176.96,30.83
S$18608
  Bottom 0.635: 170.3,27.38 165.99,31.68
S$18609
  Bottom 0.635: 163.47,7.51 163.47,7.69
S$18610
  Bottom 0.635: 163.47,7.69 170.3,14.52
S$18611
  Bottom 0.635: 170.3,14.52 170.3,27.38
S$18612
  Bottom 0.635: 198.95,36.38 197.14,36.38
S$18613
  Bottom 0.635: 197.14,36.38 192.44,31.69
S$18614
  Bottom 0.635: 192.44,31.69 185.04,31.69
S$18615
  Bottom 0.635: 204.09,31.69 204.09,32.03
S$18616
  Bottom 0.635: 204.09,32.03 199.73,36.38
S$18617
  Bottom 0.635: 199.73,36.38 198.95,36.38
S$18618
  Bottom 0.635: 198.95,36.38 198.95,46.35
S$18619
  Bottom 0.635: 198.95,46.35 194.56,50.74
S$18620
  Bottom 0.635: 142.43,27.18 146.94,31.69
S$18621
  Bottom 0.635: 142.43,27.18 142.43,23.45
S$18622
  Bottom 0.635: 142.43,23.45 131.62,12.63
S$18623
  Bottom 0.635: 131.62,12.63 130.27,12.63
S$18624
  Bottom 0.635: 142.43,27.18 137.67,31.94
S$18625
  Bottom 0.635: 137.67,31.94 128.15,31.94
S$18626
  Bottom 0.635: 128.15,31.94 127.89,31.68
S$18627
  Bottom 0.635: 222.99,31.69 222.99,38.8
S$18628
  Bottom 0.635: 222.99,38.8 217.23,44.56
S$18629
  Bottom 0.635: 217.23,44.56 217.23,47.12
S$18630
  Bottom 0.635: 217.23,47.12 213.61,50.74
S$18631
  Bottom 0.635: 225.52,12.63 225.52,13.02
S$18632
  Bottom 0.635: 225.52,13.02 219,19.53
S$18633
  Bottom 0.635: 219,19.53 218.67,19.53
S$18634
  Bottom 0.635: 218.67,19.53 217.66,20.55
S$18635
  Bottom 0.635: 217.66,20.55 217.66,26.21
S$18636
  Bottom 0.635: 217.66,26.21 222.99,31.54
S$18637
  Bottom 0.635: 222.99,31.54 222.99,31.69
S$18638
  Bottom 0.635: 222.99,31.69 223.14,31.69
S$18639
  Bottom 0.635: 287.29,33.14 287.29,13.62
S$18640
  Bottom 0.635: 287.29,13.62 286.11,12.44
S$18641
  Bottom 0.635: 286.59,38.03 287.29,37.33
S$18642
  Bottom 0.635: 287.29,37.33 287.29,33.14
S$18643
  Bottom 0.635: 298.57,31.67 298.57,32.32
S$18644
  Bottom 0.635: 298.57,32.32 297.75,33.14
S$18645
  Bottom 0.635: 297.75,33.14 287.29,33.14
S$18646
  Bottom 0.635: 286.11,12.44 286.11,11.06
S$18647
  Bottom 0.635: 286.11,11.06 286.83,10.33
S$18648
  Bottom 0.635: 286.83,10.33 296.85,10.33
S$18649
  Bottom 0.635: 296.85,10.33 298.56,12.05
S$18650
  Bottom 0.635: 298.56,12.05 298.56,12.62
S$18651
  Bottom 0.635: 280.28,12.62 280.46,12.44
S$18652
  Bottom 0.635: 280.46,12.44 286.11,12.44
S$18653
  Bottom 0.635: 258.86,31.68 249.34,22.16
S$18654
  Bottom 0.635: 249.34,22.16 249.34,12.63
S$18655
  Bottom 0.635: 263.62,50.73 257.95,45.06
S$18656
  Bottom 0.635: 257.95,45.06 257.95,32.59
S$18657
  Bottom 0.635: 257.95,32.59 258.86,31.68
S$18658
  Bottom 0.635: 92.08,7.43 76.24,23.28
S$18659
  Bottom 0.635: 76.24,23.28 76.24,26.18
S$18660
  Bottom 0.635: 76.24,26.18 70.74,31.68
S$18661
  Bottom 0.635: 266,88.83 264.62,87.45
S$18662
  Bottom 0.635: 264.62,87.45 247.5,87.45
S$18663
  Bottom 0.635: 247.5,87.45 245.83,89.13
S$18664
  Bottom 0.635: 245.83,89.13 237.72,89.13
S$18665
  Bottom 0.635: 237.72,89.13 237.43,88.83
S$18666
  Bottom 0.635: 294.56,90.21 297.82,90.21
S$18667
  Bottom 0.635: 297.82,90.21 298.56,89.47
S$18668
  Bottom 0.635: 298.56,89.47 298.56,88.82
S$18669
  Bottom 0.635: 284.23,83.42 284.23,85.28
S$18670
  Bottom 0.635: 284.23,85.28 289.15,90.21
S$18671
  Bottom 0.635: 289.15,90.21 294.56,90.21
S$18672
  Bottom 0.635: 294.56,90.21 294.56,82.84
S$18673
  Bottom 0.635: 294.56,82.84 299.32,78.08
S$18674
  Bottom 0.635: 299.32,78.08 299.32,69.77
S$18675
  Bottom 0.635: 317.61,12.62 318.37,12.62
S$18676
  Bottom 0.635: 284.23,83.42 284.62,83.42
S$18677
  Bottom 0.635: 282.19,76.81 282.19,81.67
S$18678
  Bottom 0.635: 282.19,81.67 283.94,83.42
S$18679
  Bottom 0.635: 283.94,83.42 284.23,83.42
S$18680
  Bottom 0.635: 270.76,69.78 276.19,75.21
S$18681
  Bottom 0.635: 276.19,75.21 276.19,76.81
S$18682
  Bottom 0.635: 276.19,76.81 282.19,76.81
S$18683
  Bottom 0.635: 282.4,76.81 282.19,76.81
S$18684
  Bottom 0.635: 283.78,76.81 282.4,76.81
S$18685
  Bottom 0.381: 296.75,38.03 300.61,34.17
S$18686
  Bottom 0.381: 300.61,34.17 300.61,25.76
S$18687
  Bottom 0.381: 300.61,25.76 298.17,23.31
S$18688
  Bottom 0.381: 298.17,23.31 298.17,21.96
S$18689
  Bottom 0.381: 298.17,21.96 289.76,13.55
S$18690
  Bottom 0.381: 289.76,13.55 289.76,11.6
S$18691
  Bottom 0.381: 269.52,11.6 261.31,3.38
S$18692
  Bottom 0.381: 261.31,3.38 246.77,3.38
S$18693
  Bottom 0.381: 246.77,3.38 238.56,11.6
S$18694
  Bottom 0.381: 276.98,12.62 276.98,13.89
S$18695
  Bottom 0.381: 276.98,13.89 275.24,15.63
S$18696
  Bottom 0.381: 275.24,15.63 275.24,15.88
S$18697
  Bottom 0.381: 107.58,42.08 113.05,42.08
S$18698
  Bottom 0.381: 113.05,42.08 114.55,40.57
S$18699
  Bottom 0.381: 275.71,2.46 271.04,2.46
S$18700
